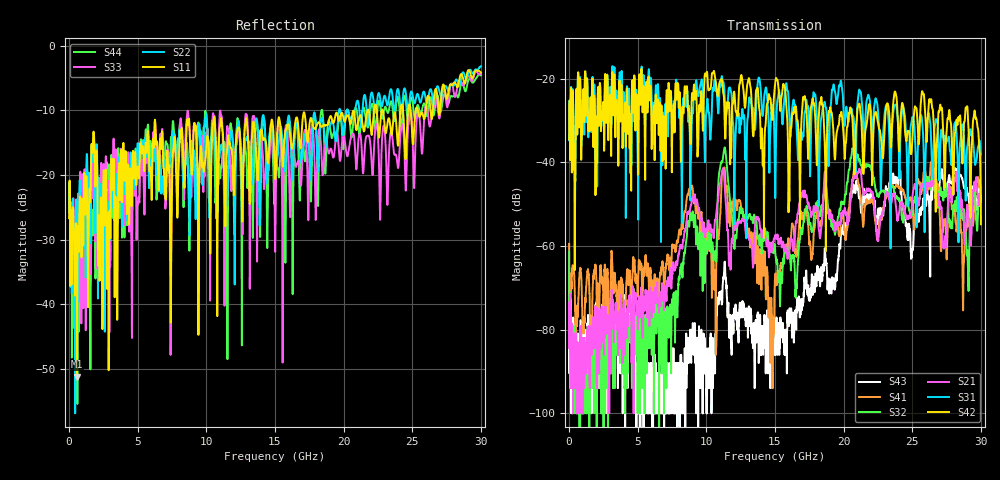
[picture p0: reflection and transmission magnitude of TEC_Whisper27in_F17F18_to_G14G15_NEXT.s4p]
! Tyco Electronics
! F17F18-G14G15_NEXT
!! PART DESCRIPTION: Whisper 27in Megtron 6 VLP-HVLP-VLP Channel Model, bulkhead 2.4mm test pts
!! MODEL DESCRIPTION: System 4-port S-parameter
!! MODEL STATUS: Measured
!! MODEL GEOMETRY: Channel Model
!! MODEL FREQUENCY RANGE: DC to 30.000 GHz in 10.000 MHz frequency steps
!! MODEL EDGE RATE LIMITATION: 12.500 ps (Using conservative 0.5/Fmax rule of thumb)
!! TIME-DOMAIN TRANSFORM CAUTIONS:
!! 1.) Do not simulate transient edge rates faster than the number listed above.  Edge rates faster than this number
!!  contain significant spectral content at frequencies above the model's highest frequency.
!! 2.) Even when simulating edge rates that are slower than the number listed above, be aware that the best time
!!  resolution possible with a direct iFFT is (1 / 2Fmax).  As a result, time resolution is typically not adequate
!!  for most time-domain simulations unless tricks such as windowing are used to minimize leakage and aliasing.
!! 3.) Because the model has a uniform frequency step, a direct iFFT will result in an impulse that that has a time
!!  length given by either (1 / Fstep) or (1 / 2Fstep), depending on the transform being used.  Care has been taken
!!  in selecting the frequency step to ensure a settled impulse response for the model.  Therefore, convolution with
!!  the model's impulse response should present no issues.  However, if directly concatenating s-parameter models
!!  in the frequency domain a user must either interpolate necessary interim frequencies or complete impulse response
!!  zero-padding.  Impulse response zero-padding is more difficult, but more accurate.
!! PORT DEFINITIONS:
!! Port  1  ----->  Side A  F17  G14  Side A  <-----  Port  2
!! Port  3  ----->  Side A  F18  G15  Side A  <-----  Port  4
! Point-to-Point link (differential)  !
! Connectors:  !
!  1: STRADA Whisper  !
! Materials:  !
!  Backplane: Megtron-6 HVLP  !
!  Daughtercard: Megtron-6 VLP  !
! Stack-up:  !
!  Backplane: 20 layers, 200mil thick  !
!  Daughtercard: 14 layers, 110mil thick  !
! Trace Length:  !
!  Backplane: 17in  !
!  Daightercards: 5in  !
! Trace Width:  !
!  Backplane: 8-13-8 mils  !
!  Daughtercards: 6-9-6 mils  !
! Geometry:  !
!  Backplane: Stripline  !
!  Daughtercards: Stripline  !
! Freq. Range: 0 GHz - 30 GHz  !
! Note1: non-mixed-mode s-parameters  !
! Note2: channel includes 2.4mm test points  !
! Touchstone data converted from IdEM dataset
# GHz S MA R 50
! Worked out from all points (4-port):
!   3000 points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, 10 MHz to 30 GHz, reference 50 ohm
!   strongest paths, dB at 10 MHz, 7.51 GHz, 15.01 GHz, 22.51 GHz, 30 GHz:
!     S42: -34.5, -34.3, -21.3, -30.6, -54.8
!     S31: -34.7, -31.1, -46.6, -27.9, -38.1
!     S21: -73.6, -66.6, -57.6, -58.2, -49.3
!     S32: -61.3, -74.9, -60.8, -48.0, -49.5
!     S41: -59.5, -60.0, -68.2, -57.6, -49.3
!     S43: -68.0, -84.4, -86.0, -52.7, -49.1
!   lowest |S11| = -51.2 dB at 590 MHz (marker M1), VSWR 1.01, Z = 49.8 - j0.119 ohm
!   |S11| at or under -10 dB: start of sweep to 21.75 GHz; 22.85 GHz to 24.14 GHz (1.291 GHz wide, 5.5 % of centre); 25.41 GHz to 25.98 GHz (573.4 MHz wide, 2.23 % of centre)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
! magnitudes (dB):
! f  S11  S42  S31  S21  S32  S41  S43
! 10 MHz  -26.7  -34.5  -34.7  -73.6  -61.3  -59.5  -68.0
! 590 MHz  -51.2  -30.9  -30.7  -100.0  -90.5  -79.2  -90.5
! 7.17 GHz  -16.4  -27.0  -28.0  -68.2  -75.9  -62.0  -94.0
! 11.31 GHz  -20.3  -26.3  -22.5  -43.9  -36.7  -41.2  -64.9
! 14.78 GHz  -11.4  -29.1  -26.3  -60.9  -59.4  -76.5  -80.0
! 20.79 GHz  -10.6  -42.9  -32.5  -43.6  -37.7  -42.4  -45.5
! 30 GHz  -4.2  -54.8  -38.1  -49.3  -49.5  -49.3  -49.1
